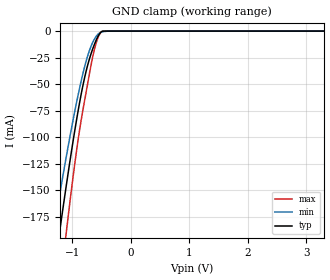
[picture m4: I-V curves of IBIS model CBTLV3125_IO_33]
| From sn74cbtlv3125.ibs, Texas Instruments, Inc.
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[Model]   CBTLV3125_IO_33
Model_type  Terminator
| variable   typ   min   max
C_comp   5.05pF   4.23pF   5.80pF
| C_tri-state   5.05pF   4.23pF   5.80pF
[Temperature Range]   40   100   -40
| Ambient temperature   25   85   -40
[Voltage range]   3.3   3   3.6
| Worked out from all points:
|   GND clamp passes 1 mA (typ) near -0.51 V on its own axis
[GND Clamp]
| CBTLV3125_IO_33
|   Voltage   I(typ)   I(min)   I(max)
-3.3V     -1.111A    -924.3mA   -1.39A
-1.315V   -229.3mA   -187.7mA   -294.7mA
-1.215V   -189.6mA   -154.8mA   -245mA
-1.1V     -145.6mA   -118.4mA   -189.7mA
-910mV    -79.02mA   -63.39mA   -107mA
-845mV    -59.31mA   -46.89mA   -83.71mA
-775mV    -41.03mA   -31.21mA   -61.77mA
-700mV    -25.44mA   -17.64mA   -38.86mA
-620mV    -12.61mA   -7.609mA   -17.33mA
-555mV    -4.639mA   -2.778mA   -5.769mA
-490mV    -337uA     -838.1uA   -335.4uA
3.3V      1.318nA    61.76nA    17.3pA
